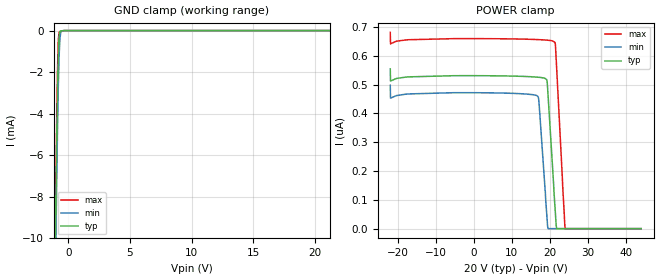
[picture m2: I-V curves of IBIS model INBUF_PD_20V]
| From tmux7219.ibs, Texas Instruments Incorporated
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| Model4
[Model]   INBUF_PD_20V
Model_type   Input
Vinl = 0.8
Vinh = 1.3
|   typ   min   max
C_comp   1.85pF   1.7pF   2.1pF
[Voltage Range]   20   18   22
[Temperature Range]   27   130   -40
[Power Clamp Reference]   20   18   22
[GND Clamp Reference]   0   0   0
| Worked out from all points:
|   GND clamp passes 1 mA (typ) near -0.80 V on its own axis
[GND Clamp]
|   Voltage   I(typ)   I(min)   I(max)
-22V      -1.138A    -1.136A    -1.139A
-1.078V   -11.61mA   -13.22mA   -10.52mA
-1.012V   -8.543mA   -10.23mA   -7.394mA
-946mV    -5.661mA   -7.404mA   -4.464mA
-880mV    -3.122mA   -4.849mA   -1.972mA
-814mV    -1.239mA   -2.735mA   -452.2uA
-748mV    -285.6uA   -1.241mA   -78.59uA
-682mV    -51.81uA   -399.5uA   -43.07uA
-616mV    -20.92uA   -87.62uA   -29.75uA
-550mV    -11.66uA   -20.66uA   -18.41uA
-154mV    0A         0A         0A
44V       0A         0A         0A
[POWER Clamp]
|   Voltage   I(typ)   I(min)   I(max)
-22V      554.3nA    497.7nA    681nA
-21.93V   512.1nA    452.8nA    641.2nA
16.74V    525.6nA    460nA      656.1nA
17.14V    525.2nA    433.7nA    655.9nA
19.12V    517.6nA    57.01nA    654.2nA
19.51V    460.1nA    0A         653.8nA
21.3V     80.51nA    0A         646.5nA
21.43V    54.5nA     0A         638nA
21.76V    0A         0A         558nA
23.94V    0A         0A         4.783nA
24.07V    0A         0A         0A
44V       0A         0A         0A
